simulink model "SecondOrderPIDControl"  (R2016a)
settings: Solver=VariableStepAuto  StartTime=0.0  StopTime=Tf  RelTol=1e-7  AbsTol=1e-6
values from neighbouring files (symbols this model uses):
  d = 0    [Section4p2_DCMotorOpenLoop.m]    (also in Section4p3_DCMotorPControl.m; Section4p4_DCMotorPIControl.m; Section4p5_RocketPDControl.m = -0.01; Section4p6_PIDSecondOrder.m = 2)
  Gden = [1 a0]    [Section4p2_DCMotorOpenLoop.m]    (also in Section4p3_DCMotorPControl.m = [J*L (J*R+b*L) (Kt*Ke+b*R)]; Section4p4_DCMotorPIControl.m; Section4p5_RocketPDControl.m = [1 a1 a0]; Section4p6_PIDSecondOrder.m = [1 a1 a0])
  Gnum = b0    (= 766.8)    [Section4p2_DCMotorOpenLoop.m]    (also in Section4p3_DCMotorPControl.m = 0.00122680374957; Section4p4_DCMotorPIControl.m; Section4p5_RocketPDControl.m = 6.32; Section4p6_PIDSecondOrder.m = 17)
  Kd = (2*zeta*wn-a1)/b0    [Section4p5_RocketPDControl.m]    (also in Section4p6_PIDSecondOrder.m = 1)
  Ki = Kp/2    (= 0.001)    [Section4p4_DCMotorPIControl.m]    (also in Section4p6_PIDSecondOrder.m = 15.006002401; Section4p6_PIFirstOrder.m = 10.8843537415)
  Kp = 16    [Section4p3_DCMotorPControl.m]    (also in Section4p4_DCMotorPIControl.m = 0.002; Section4p5_RocketPDControl.m = (wn^2-a0)/b0; Section4p6_PIDSecondOrder.m = 4.94237695078; Section4p6_PIFirstOrder.m = 2)
  r = 1000    [Section4p2_DCMotorOpenLoop.m]    (also in Section4p3_DCMotorPControl.m; Section4p4_DCMotorPIControl.m; Section4p5_RocketPDControl.m = 0.1; Section4p6_PIDSecondOrder.m = 4)
  Tf = 5    [Section4p2_DCMotorOpenLoop.m]    (also in Section4p3_DCMotorPControl.m = 0.005; Section4p4_DCMotorPIControl.m = 10; Section4p5_RocketPDControl.m = 10; Section4p6_PIDSecondOrder.m = 4)

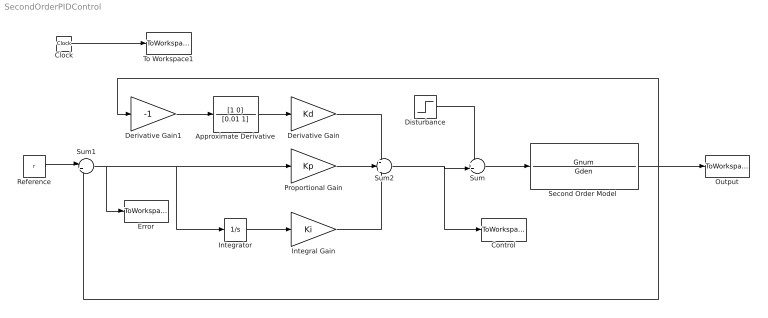
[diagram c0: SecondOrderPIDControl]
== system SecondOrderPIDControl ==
  Approximate Derivative : TransferFcn  Numerator=[1 0]  Denominator=[0.01 1]
  Clock : Clock
  Control : ToWorkspace  VariableName=u  SampleTime=-1
  Derivative Gain : Gain  Gain=Kd
  Derivative Gain1 : Gain  Gain=-1
  Disturbance : Step  Time=Tf/2  After=d  SampleTime=0
  Error : ToWorkspace  VariableName=e  SampleTime=-1
  Integral Gain : Gain  Gain=Ki
  Integrator : Integrator
  Output : ToWorkspace  VariableName=y  SampleTime=-1
  Proportional Gain : Gain  Gain=Kp
  Reference : Constant  Value=r
  "Second Order Model " : TransferFcn  Numerator=Gnum  Denominator=Gden
  Sum : Sum  Inputs=++|
  Sum1 : Sum  Inputs=|+-
  Sum2 : Sum  Inputs=+++
  To Workspace1 : ToWorkspace  VariableName=t  SampleTime=-1
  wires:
  Clock/1 -> To Workspace1/1
  Disturbance/1 -> Sum/1
  Sum/1 -> "Second Order Model "/1
  Reference/1 -> Sum1/1
  Sum1/1 -> Error/1, Proportional Gain/1, Integrator/1
  Sum2/1 -> Sum/2, Control/1
  Integrator/1 -> Integral Gain/1
  Integral Gain/1 -> Sum2/3
  Proportional Gain/1 -> Sum2/2
  Derivative Gain/1 -> Sum2/1
  Approximate Derivative/1 -> Derivative Gain/1
  Derivative Gain1/1 -> Approximate Derivative/1
  "Second Order Model "/1 -> Derivative Gain1/1, Sum1/2, Output/1
